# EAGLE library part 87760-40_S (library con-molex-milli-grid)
HEADER
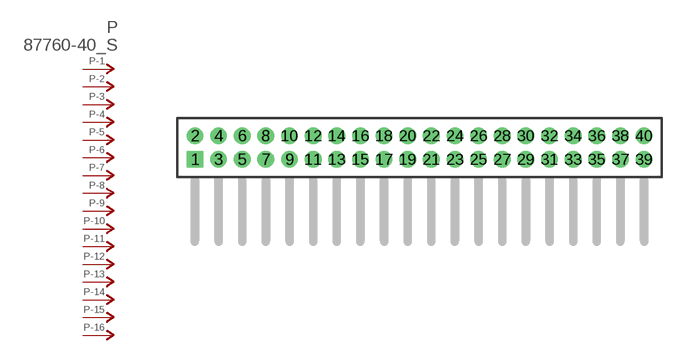
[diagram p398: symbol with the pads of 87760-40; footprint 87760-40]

Designator prefix P; gates -1=P-NV -2=P-N -3=P-N -4=P-N -5=P-N -6=P-N -7=P-N -8=P-N -9=P-N -10=P-N -11=P-N -12=P-N -13=P-N -14=P-N -15=P-N -16=P-N -17=P-N -18=P-N -19=P-N -20=P-N -21=P-N -22=P-N -23=P-N -24=P-N -25=P-N -26=P-N -27=P-N -28=P-N -29=P-N -30=P-N -31=P-N -32=P-N -33=P-N -34=P-N -35=P-N -36=P-N -37=P-N -38=P-N -39=P-N -40=P-N

## 87760-40_S  [87760-40]
1  -1:P  pas
2  -2:P  pas
3  -3:P  pas
4  -4:P  pas
5  -5:P  pas
6  -6:P  pas
7  -7:P  pas
8  -8:P  pas
9  -9:P  pas
10  -10:P  pas
11  -11:P  pas
12  -12:P  pas
13  -13:P  pas
14  -14:P  pas
15  -15:P  pas
16  -16:P  pas
17  -17:P  pas
18  -18:P  pas
19  -19:P  pas
20  -20:P  pas
21  -21:P  pas
22  -22:P  pas
23  -23:P  pas
24  -24:P  pas
25  -25:P  pas
26  -26:P  pas
27  -27:P  pas
28  -28:P  pas
29  -29:P  pas
30  -30:P  pas
31  -31:P  pas
32  -32:P  pas
33  -33:P  pas
34  -34:P  pas
35  -35:P  pas
36  -36:P  pas
37  -37:P  pas
38  -38:P  pas
39  -39:P  pas
40  -40:P  pas

## Footprint 87760-40 (pad centres in mm)
HEADER Dual Row, Right Angle
drill 0.914 square: 1 -19,-1
drill 0.914: 2 -19,1; 3 -17,-1; 4 -17,1; 5 -15,-1; 6 -15,1; 7 -13,-1; 8 -13,1; 9 -11,-1; 10 -11,1; 11 -9,-1; 12 -9,1; 13 -7,-1; 14 -7,1; 15 -5,-1; 16 -5,1; 17 -3,-1; 18 -3,1; 19 -1,-1; 20 -1,1; 21 1,-1; 22 1,1; 23 3,-1; 24 3,1; 25 5,-1; 26 5,1; 27 7,-1; 28 7,1; 29 9,-1; 30 9,1; 31 11,-1; 32 11,1; 33 13,-1; 34 13,1; 35 15,-1; 36 15,1; 37 17,-1; 38 17,1; 39 19,-1; 40 19,1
